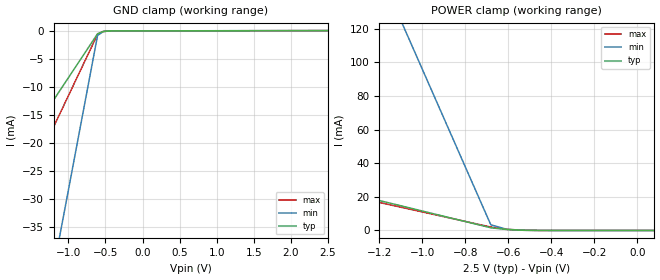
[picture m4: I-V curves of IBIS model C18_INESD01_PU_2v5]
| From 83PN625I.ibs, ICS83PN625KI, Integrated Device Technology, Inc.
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[Model] C18_INESD01_PU_2v5
Model_type   Input
Polarity   Non-Inverting
Vinl = 0.7V
Vinh = 1.7V
|   typ   min   max
C_comp   2pF   1.5pF   2.5pF
|   typ   min   max
[Voltage range]   2.5V   2.375V   2.625V
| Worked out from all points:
|   GND clamp passes 1 mA (typ) near -0.63 V on its own axis
|   POWER clamp passes 1 mA (typ) near -0.64 V on its own axis
[GND_clamp]
|Voltage   I (typ)   I (min)   I (max)
-2.5V     -38.24mA   -133.4mA   -53.3mA
-2.424V   -36.73mA   -128.1mA   -51.19mA
-2.348V   -35.23mA   -122.8mA   -49.08mA
-1.894V   -26.18mA   -90.98mA   -36.45mA
-1.818V   -24.68mA   -85.68mA   -34.35mA
-1.136V   -11.11mA   -37.97mA   -15.4mA
-1.061V   -9.604mA   -32.67mA   -13.29mA
-606.1mV  -561.5uA   -857.1uA   -660.6uA
-530.3mV  -155.4uA   -179.8uA   -155.3uA
-454.5mV  -73.25uA   -73.73uA   -74.15uA
2.5V      8.386pA    2.339uA    653.8nA
[Power_clamp]
|Voltage   I (typ)   I (min)   I (max)
-2.5V     58.46mA    531.7mA    53.33mA
-1.136V   15.82mA    135.5mA    14.86mA
-1.061V   13.45mA    113.4mA    12.72mA
-681.8mV  1.609mA    3.381mA    2.038mA
-606.1mV  556uA      651uA      681uA
-530.3mV  127.1uA    136.6uA    130.1uA
75.76mV   -1.514uA   -1.417uA   -1.608uA
